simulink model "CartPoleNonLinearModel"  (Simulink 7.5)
settings: Solver=ode45  StartTime=0.0  StopTime=10.0  RelTol=1e-3
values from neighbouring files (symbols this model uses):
  g = 9.81    [Esercitazione09.m]
  L = 1    [Esercitazione09.m]
  m = 0.1    [Esercitazione09.m]
  M = 1    [Esercitazione09.m]
  X0 = [1 0 0.55 0]'    [Esercitazione09.m]

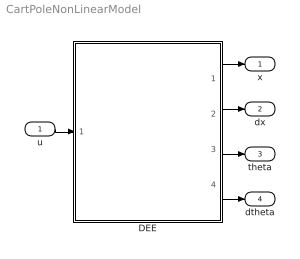
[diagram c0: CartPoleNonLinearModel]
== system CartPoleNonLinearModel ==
  u : Inport  OutDataType=fixdt(1, 16)  OutScaling=2^0
  DEE : Subsystem
  x : Outport  OutDataType=fixdt(1, 16)  OutScaling=2^0
  dx : Outport  Port=2  OutDataType=fixdt(1, 16)  OutScaling=2^0
  theta : Outport  Port=3  OutDataType=fixdt(1, 16)  OutScaling=2^0
  dtheta : Outport  Port=4  OutDataType=fixdt(1, 16)  OutScaling=2^0
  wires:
  u/1 -> DEE/1(SysInport1)
  DEE/1(Port1) -> x/1
  DEE/2(Port2) -> dx/1
  DEE/3(Port3) -> theta/1
  DEE/4(Port4) -> dtheta/1

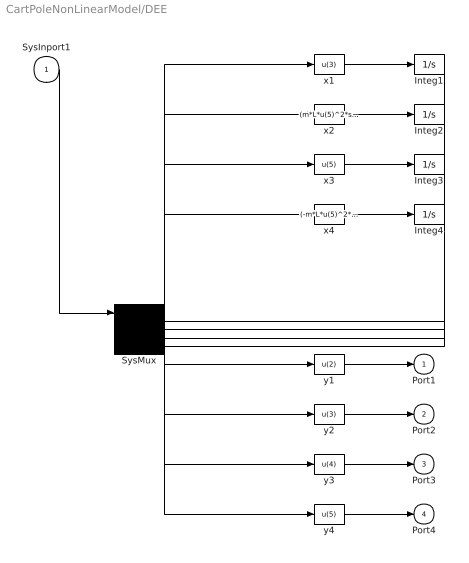
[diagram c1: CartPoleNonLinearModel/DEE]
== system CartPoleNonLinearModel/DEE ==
  SysInport1 : Inport
  Integ1 : Integrator  InitialCondition=X0(1)
  Integ2 : Integrator  InitialCondition=X0(2)
  Integ3 : Integrator  InitialCondition=X0(3)
  Integ4 : Integrator  InitialCondition=X0(4)
  SysMux : Mux  Inputs=5
  x1 : Fcn  Expr=u(3)
  x2 : Fcn  Expr=(m*L*u(5)^2*sin(u(4)) - m*g*sin(u(4))*cos(u(4))+ u)/(M+m*sin(u(4))^2)
  x3 : Fcn  Expr=u(5)
  x4 : Fcn  Expr=(-m*L*u(5)^2*sin(u(4))*cos(u(4))+(M+m)*g*sin(u(4))-u*cos(u(4)))/((M+m*sin(u(4))^2)*L)
  y1 : Fcn  Expr=u(2)
  y2 : Fcn  Expr=u(3)
  y3 : Fcn  Expr=u(4)
  y4 : Fcn  Expr=u(5)
  Port1 : Outport
  Port2 : Outport  Port=2
  Port3 : Outport  Port=3
  Port4 : Outport  Port=4
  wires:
  SysInport1/1 -> SysMux/1
  SysMux/1 -> x1/1, x2/1, x3/1, x4/1, y1/1, y2/1, y3/1, y4/1
  x1/1 -> Integ1/1
  Integ1/1 -> SysMux/2
  x2/1 -> Integ2/1
  Integ2/1 -> SysMux/3
  x3/1 -> Integ3/1
  Integ3/1 -> SysMux/4
  x4/1 -> Integ4/1
  Integ4/1 -> SysMux/5
  y1/1 -> Port1/1
  y2/1 -> Port2/1
  y3/1 -> Port3/1
  y4/1 -> Port4/1
